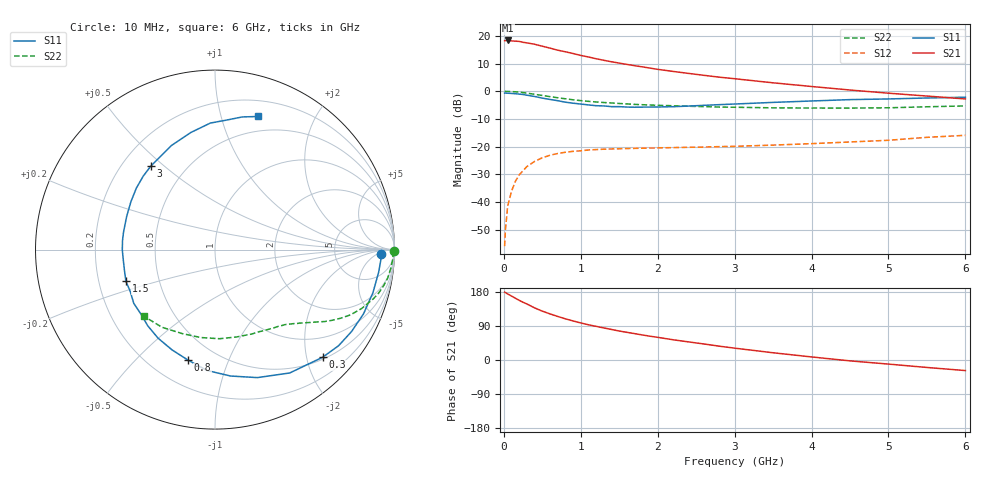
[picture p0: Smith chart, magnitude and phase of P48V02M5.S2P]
! SIEMENS Small Signal Semiconductors
! BFP182
! Si NPN RF Bipolar Junction Transistor in SOT143
! VCE = 8 V  IC = 2.5 mA
! Common Emitter S-Parameters:  March  1996
# GHz  S  MA  R  50
!  f  S11  S21  S12  S22
! GHz  MAG  ANG  MAG  ANG  MAG  ANG  MAG  ANG
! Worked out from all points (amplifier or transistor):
!   36 points, 10 MHz to 6 GHz, reference 50 ohm
!   highest |S21| = 18.3 dB at 50 MHz (marker M1)
!   |S21| within 3 dB of that: start of sweep to 632.2 MHz
!   unconditionally stable (mu >= 1): 2.105 GHz to 5.928 GHz
!   at 250 MHz: K = 0.14, MSG = 23.2 dB, |S12| = -28.7 dB
!   at 1.4 GHz: K = 0.72, MSG = 15.7 dB, |S12| = -20.8 dB
!   at 6 GHz: K = 0.99, MSG = 6.6 dB, |S12| = -15.9 dB
!   S11 on the Smith chart (normalised r, x): 10 MHz: 24, -8; 300 MHz: 0.54, -2.31; 800 MHz: 0.35, -0.72; 1.5 GHz: 0.32, -0.15; 3 GHz: 0.32, +0.45; 6 GHz: 0.35, +1.31
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0.01  0.9269 -1.5  8.157 179.0  0.0016 83.9  0.9947 -0.6
0.02  0.9265 -3.2  8.185 178.1  0.0031 88.5  0.9922 -1.3
0.05  0.9204 -7.9  8.239 174.3  0.0085 88.1  0.9918 -3.1
0.1  0.9121 -15.3  8.087 168.7  0.0157 80.5  0.9845 -6.2
0.2  0.8872 -31.0  7.922 157.4  0.031 72.3  0.9608 -12.1
0.3  0.8482 -45.0  7.445 147.8  0.0438 64.8  0.9234 -17.3
0.4  0.8036 -58.8  7.039 137.5  0.0541 57.5  0.8805 -21.9
0.5  0.7512 -71.7  6.487 128.9  0.063 51.0  0.838 -25.7
0.6  0.7096 -83.0  5.997 121.7  0.07 46.0  0.7984 -28.6
0.7  0.675 -93.7  5.501 115.0  0.0752 42.0  0.7624 -31.1
0.8  0.6339 -103.7  5.15 108.6  0.0792 38.0  0.7302 -33.3
1  0.5867 -122.7  4.425 97.8  0.0841 32.0  0.6765 -36.8
1.1  0.5661 -131.5  4.145 92.9  0.0871 29.9  0.6562 -38.3
1.3  0.5427 -146.5  3.61 84.6  0.09 26.2  0.6252 -40.9
1.5  0.5267 -160.5  3.217 76.5  0.0914 23.7  0.6004 -43.4
1.8  0.5164 -179.8  2.752 66.1  0.0937 21.5  0.571 -47.1
2.2  0.5257 159.4  2.276 53.4  0.096 19.5  0.5466 -52.8
3  0.5872 127.4  1.681 31.3  0.1013 18.4  0.5134 -66.2
3.5  0.6287 112.7  1.417 19.1  0.1066 18.4  0.5015 -76.0
4.5  0.7055 92.1  1.051 -2.3  0.1215 18.6  0.4962 -99.1
5.5  0.7545 78.4  0.818 -19.7  0.1472 17.6  0.5238 -124.3
6  0.7789 72.2  0.725 -27.9  0.16 14.4  0.5427 -136.7
